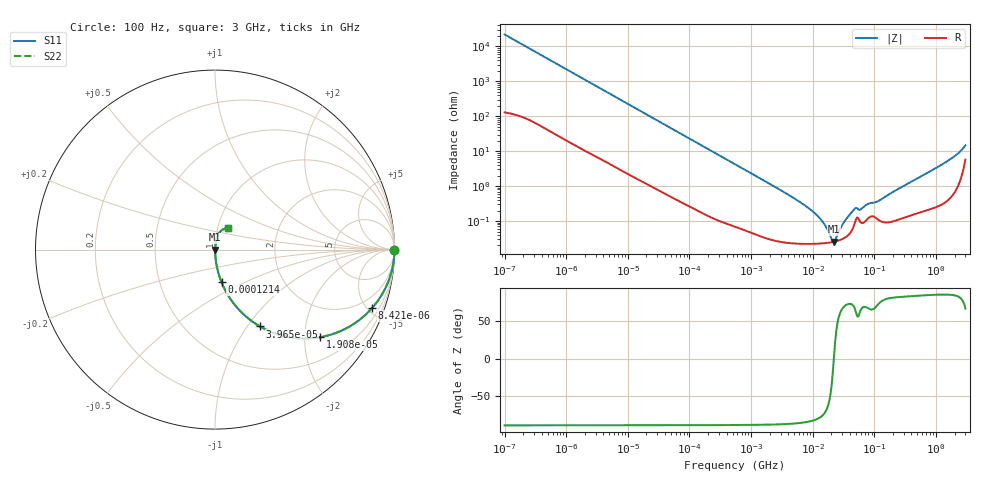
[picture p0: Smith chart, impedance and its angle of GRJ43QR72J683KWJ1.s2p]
!Murata Part Number: GRJ43QR72J683KWJ1
!These Parameters are Measured in Series Mode Connection
!Data Generated on Jun 19, 2026
!  o--ll--o
!Port1  Port2
!  o------o
!Operation Temp=25[degC], DC Bias Voltage=0[V]
!Freq. Start=100[Hz] Stop=3[GHz] 401[Steps]
# Hz S RI R 50
!Freq.(Hz) S11(Real) S11(Imag) S21(Real) S21(Imag) S12(Real) S12(Imag) S22(Real) S22(Imag)
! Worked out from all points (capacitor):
!   401 points, 100 Hz to 3 GHz, reference 50 ohm
!   read as one part in series: C = 72.3 nF near 109 Hz
!   lowest |Z| = 25.7 mohm at 22.19 MHz (marker M1)
!   series resonance near 21.99 MHz, so ESL is about 720 pH
!   S11 on the Smith chart (normalised r, x): 100 Hz: open; 8.421 kHz: 1.05, -5.36; 19.08 kHz: 1.02, -2.38; 39.66 kHz: 1.01, -1.15; 121.4 kHz: 1.00, -0.38; 3 GHz: 1.12, +0.27
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100  1 -0.00455  4.74e-05 0.00455  4.74e-05 0.00455  1 -0.00455
1788  0.9929 -0.0793  0.00707 0.0793  0.00707 0.0793  0.9929 -0.0793
4610  0.958 -0.1959  0.042 0.1959  0.042 0.1959  0.958 -0.1959
8421  0.8755 -0.3253  0.1245 0.3253  0.1245 0.3253  0.8755 -0.3253
19078  0.5851 -0.4876  0.4149 0.4876  0.4149 0.4876  0.5851 -0.4876
31977  0.3381 -0.4679  0.6619 0.4679  0.6619 0.4679  0.3381 -0.4679
39655  0.2508 -0.4282  0.7492 0.4282  0.7492 0.4282  0.2508 -0.4282
66468  0.1086 -0.3057  0.8914 0.3057  0.8914 0.3057  0.1086 -0.3057
121426  0.0365 -0.1819  0.9635 0.1819  0.9635 0.1819  0.0365 -0.1819
547723  0.00247 -0.0422  0.9975 0.0422  0.9975 0.0422  0.00247 -0.0422
4141163  0.000264 -0.00548  0.9997 0.00548  0.9997 0.00548  0.000264 -0.00548
9794414  0.000226 -0.00193  0.9998 0.00193  0.9998 0.00193  0.000226 -0.00193
1.442825e7  0.00023 -0.000935  0.9998 0.000935  0.9998 0.000935  0.00023 -0.000935
2.035898e7  0.000248 -0.000168  0.9998 0.000168  0.9998 0.000168  0.000248 -0.000168
2.21892e7  0.000256 1.97e-05  0.9997 -1.97e-05  0.9997 -1.97e-05  0.000256 1.97e-05
2.418395e7  0.000266 0.000208  0.9997 -0.000208  0.9997 -0.000208  0.000266 0.000208
3.268714e7  0.000329 0.000913  0.9997 -0.000913  0.9997 -0.000913  0.000329 0.000913
4.612319e7  0.000706 0.00197  0.9993 -0.00197  0.9993 -0.00197  0.000706 0.00197
5.9714e7  0.000921 0.00194  0.9991 -0.00194  0.9991 -0.00194  0.000921 0.00194
1.751444e8  0.000957 0.00581  0.999 -0.00581  0.999 -0.00581  0.000957 0.00581
1.443257e9  0.00583 0.0481  0.9942 -0.0481  0.9942 -0.0481  0.00583 0.0481
3e9  0.0697 0.1194  0.9303 -0.1194  0.9303 -0.1194  0.0697 0.1194
